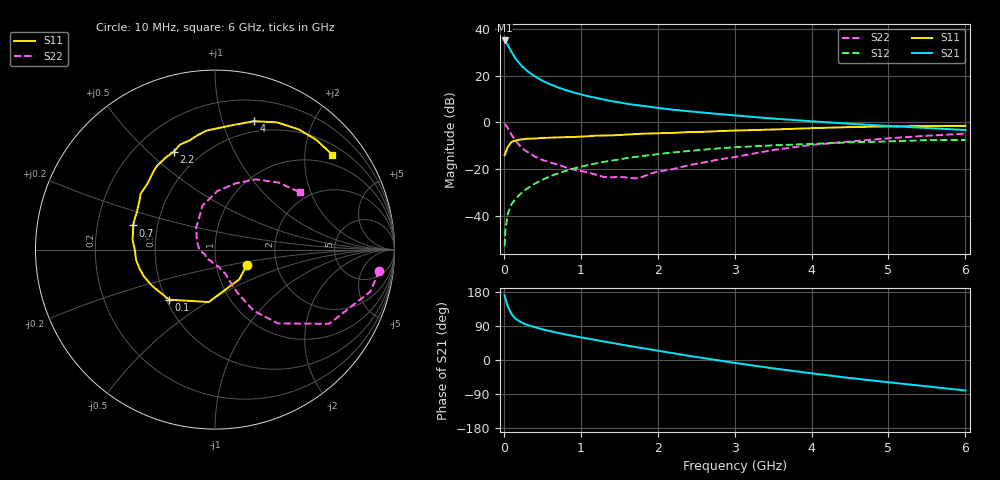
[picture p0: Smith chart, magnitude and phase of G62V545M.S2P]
! SIEMENS Small Signal Semiconductors
! BFG193
! Si NPN RF Bipolar Junction Transistor in SOT223
! VCE = 2.5 V  IC = 45 mA
! Common Emitter S-Parameters:  August  1996
# GHz  S  MA  R  50
!  f  S11  S21  S12  S22
! GHz  MAG  ANG  MAG  ANG  MAG  ANG  MAG  ANG
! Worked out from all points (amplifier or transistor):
!   36 points, 10 MHz to 6 GHz, reference 50 ohm
!   highest |S21| = 35.1 dB at 10 MHz (marker M1)
!   |S21| within 3 dB of that: start of sweep to 68.32 MHz
!   unconditionally stable (mu >= 1): 396.9 MHz to 2.466 GHz
!   at 250 MHz: K = 0.91, MSG = 26.7 dB, |S12| = -29.7 dB
!   at 1.4 GHz: K = 1.05, MAG = 11.4 dB, |S12| = -16.5 dB
!   at 6 GHz: K = 0.91, MSG = 2.1 dB, |S12| = -7.6 dB
!   S11 on the Smith chart (normalised r, x): 10 MHz: 1.40, -0.26; 100 MHz: 0.52, -0.34; 700 MHz: 0.36, +0.13; 2.2 GHz: 0.36, +0.60; 4 GHz: 0.39, +1.27; 6 GHz: 0.73, +2.64
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0.01  0.1964 -26.6  56.96 170.8  0.0022 86.0  0.9229 -7.3
0.02  0.2138 -50.6  54.71 162.9  0.0047 75.8  0.8967 -15.1
0.05  0.2942 -96.8  45.93 141.5  0.0108 69.7  0.7587 -33.0
0.1  0.3788 -132.6  32.19 121.5  0.0176 66.2  0.54 -49.6
0.15  0.4055 -150.5  23.55 109.2  0.0224 64.2  0.4039 -57.6
0.2  0.4234 -159.4  18.53 102.4  0.0275 66.4  0.3249 -60.2
0.25  0.4337 -166.1  15.09 97.0  0.0326 66.5  0.2679 -62.5
0.3  0.4432 -172.4  12.76 92.9  0.0377 68.1  0.2346 -63.8
0.4  0.447 -179.8  9.703 86.8  0.0478 68.1  0.1852 -65.3
0.5  0.4628 173.1  7.796 81.0  0.0583 67.5  0.1557 -66.0
0.6  0.466 168.3  6.553 76.3  0.0692 66.3  0.1384 -68.0
0.7  0.4758 163.6  5.643 71.7  0.0798 65.1  0.1235 -71.7
0.9  0.4831 154.2  4.399 63.5  0.1012 61.7  0.0968 -77.8
1.1  0.5029 146.6  3.618 56.2  0.1212 58.0  0.0838 -92.1
1.6  0.5455 130.2  2.5 38.0  0.1704 46.9  0.0652 -140.8
2.2  0.5912 113.0  1.861 18.0  0.2251 33.1  0.0991 164.6
2.8  0.6466 98.2  1.502 -1.3  0.2764 18.9  0.1601 131.3
3.5  0.7002 82.0  1.202 -22.0  0.3203 1.4  0.2547 105.8
4  0.7476 73.1  1.051 -35.1  0.3433 -8.4  0.3271 87.6
4.5  0.7888 64.0  0.928 -47.6  0.3722 -18.5  0.3875 72.4
5.5  0.8321 47.3  0.755 -69.6  0.4141 -41.7  0.5149 46.5
6  0.8401 39.1  0.683 -80.5  0.4184 -55.0  0.5702 34.0
